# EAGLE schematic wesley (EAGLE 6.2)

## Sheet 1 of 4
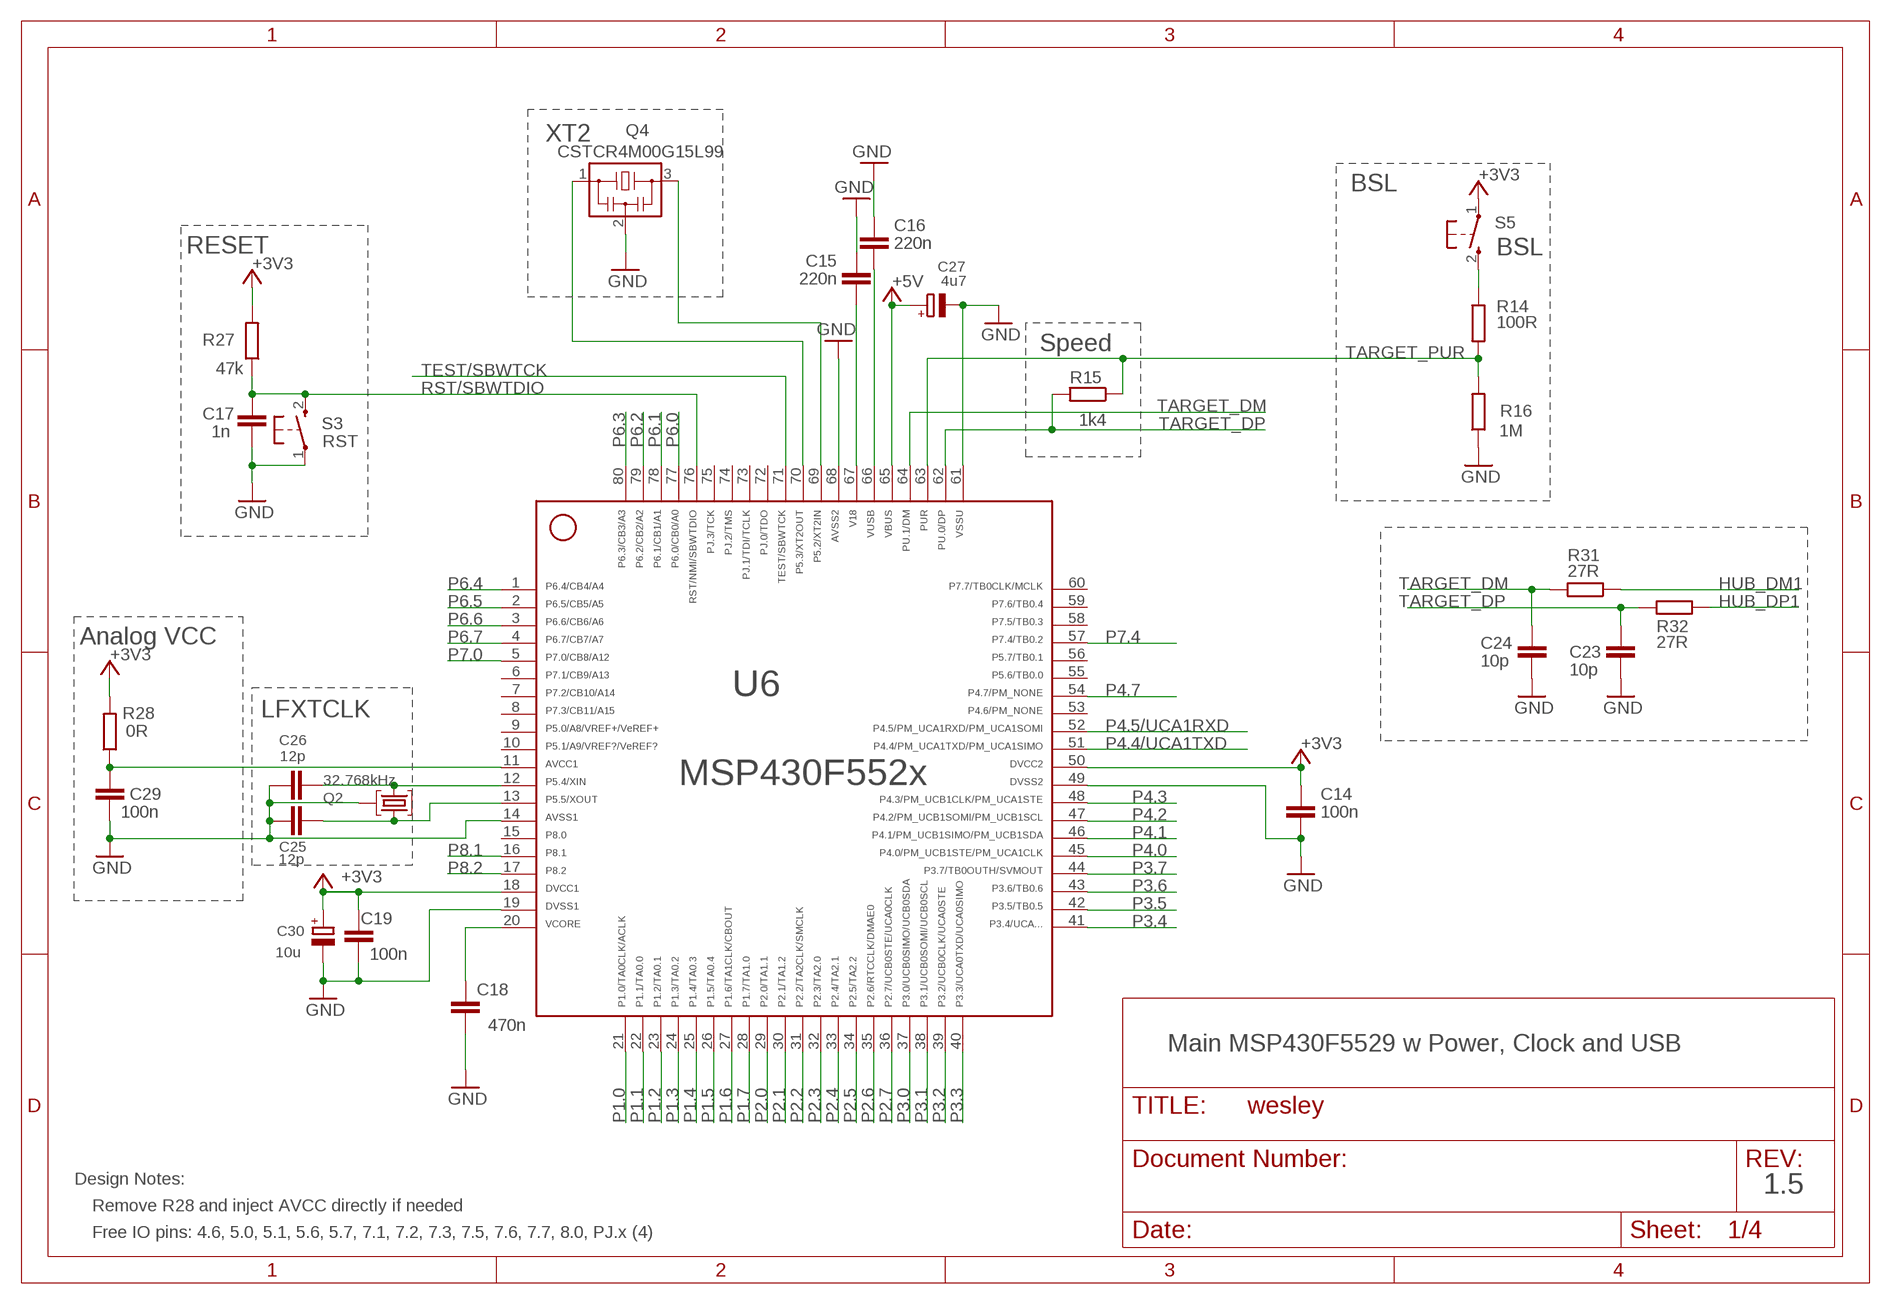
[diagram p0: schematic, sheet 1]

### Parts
C14  100n  C-EUC0402  [C0402]
C15  220n  C-EUC0402  [C0402]
C16  220n  C-EUC0402  [C0402]
C17  1n  C-EUC0402  [C0402]
C18  470n  C-EUC0402  [C0402]
C19  100n  C-EUC0402  [C0402]
C23  10p  C-EUC0402  [C0402]
C24  10p  C-EUC0402  [C0402]
C25  12p  C-EUC0402  [C0402]
C26  12p  C-EUC0402  [C0402]
C27  4u7  CPOL-EUA/3216-18R  [A/3216-18R]
C29  100n  C-EUC0402  [C0402]
C30  10u  CPOL-EUA/3216-18R  [A/3216-18R]
Q2  32.768kHz  MS3V-T1R  [MS3V-T1R]
Q4  CSTCR4M00G15L99  MURATA-FILTER_CSTCR6M00G53Z  [MURATA-FILTER_CSTCR]
R14  100R  R-EU_R0402  [R0402]
R15  1k4  R-EU_R0402  [R0402]
R16  1M  R-EU_R0402  [R0402]
R27  47k  R-EU_R0402  [R0402]
R28  0R  R-EU_R0402  [R0402]
R31  27R  R-EU_R0402  [R0402]
R32  27R  R-EU_R0402  [R0402]
S3  RST  PB  [PBTH]
S5  BSL  PB  [PBTH]
U6  MSP430F5529IPNR  F552X---PN80  [PN80]

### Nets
+3V3 [Power]: C14.1 C19.2 C30.+ R27.2 R28.2 S5.1(P) U6.18 U6.50 ; also sheet 2
+5V [Power]: C27.+ U6.65 ; also sheet 2
AVCC [Power]: C29.1 R28.1 U6.11
GND [Ground]: C14.2 C15.2 C16.2 C17.2 C18.1 C19.1 C23.2 C24.2 C25.1 C26.1 C27.- C29.2 C30.- Q2.P3(GND) Q4.2 R16.1 S3.1(P) U6.14 U6.19 U6.49 U6.61 U6.68 ; also sheet 2,3,4
HUB_DM1: R31.1 ; also sheet 4
HUB_DP1: R32.1 ; also sheet 4
N$4: R14.1 S5.2(S)
P1.0: U6.21 ; also sheet 2
P1.1: U6.22 ; also sheet 2
P1.2: U6.23 ; also sheet 2
P1.3: U6.24 ; also sheet 2
P1.4: U6.25 ; also sheet 2
P1.5: U6.26 ; also sheet 2
P1.6: U6.27 ; also sheet 2
P1.7: U6.28 ; also sheet 2
P2.0: U6.29 ; also sheet 2
P2.1: U6.30 ; also sheet 2
P2.2: U6.31 ; also sheet 2
P2.3: U6.32 ; also sheet 2
P2.4: U6.33 ; also sheet 2
P2.5: U6.34 ; also sheet 2
P2.6: U6.35 ; also sheet 2
P2.7: U6.36 ; also sheet 2
P3.0: U6.37 ; also sheet 2
P3.1: U6.38 ; also sheet 2
P3.2: U6.39 ; also sheet 2
P3.3: U6.40 ; also sheet 2
P3.4: U6.41 ; also sheet 2
P3.5: U6.42 ; also sheet 2
P3.6: U6.43 ; also sheet 2
P3.7: U6.44 ; also sheet 2
P4.0: U6.45 ; also sheet 2
P4.1: U6.46 ; also sheet 2
P4.2: U6.47 ; also sheet 2
P4.3: U6.48 ; also sheet 2
P4.4/UCA1TXD: U6.51 ; also sheet 2
P4.5/UCA1RXD: U6.52 ; also sheet 2
P4.7: U6.54 ; also sheet 2
P5.2/XT2IN: Q4.3 U6.69
P5.3/XT2OUT: Q4.1 U6.70
P5.4/XIN: C26.2 Q2.P2 U6.12
P5.5/XOUT: C25.2 Q2.P1 U6.13
P6.0: U6.77 ; also sheet 2
P6.1: U6.78 ; also sheet 2
P6.2: U6.79 ; also sheet 2
P6.3: U6.80 ; also sheet 2
P6.4: U6.1 ; also sheet 2
P6.5: U6.2 ; also sheet 2
P6.6: U6.3 ; also sheet 2
P6.7: U6.4 ; also sheet 2
P7.0: U6.5 ; also sheet 2
P7.4: U6.57 ; also sheet 2
P8.1: U6.16 ; also sheet 2
P8.2: U6.17 ; also sheet 2
RST/SBWTDIO: C17.1 R27.1 S3.2(S) U6.76 ; also sheet 2
TARGET_DM: C24.1 R31.2 U6.64
TARGET_DP: C23.1 R15.2 R32.2 U6.62
TARGET_PUR: R14.2 R15.1 R16.2 U6.63
TARGET_VUSB [Power]: C16.1 U6.66
TEST/SBWTCK: U6.71 ; also sheet 2
V18 [Power]: C15.1 U6.67
VCORE [Power]: C18.2 U6.20
Unconnected: U6.6 U6.7 U6.8 U6.9 U6.10 U6.15 U6.53 U6.55 U6.56 U6.58 U6.59 U6.60 U6.72 U6.73 U6.74 U6.75

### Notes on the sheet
- XT2
- BSL
- RESET
- Speed
- Analog VCC
- LFXTCLK
- Main MSP430F5529 w Power, Clock and USB
- Design Notes:
- 1.5
- Remove R28 and inject AVCC directly if needed
- Free IO pins: 4.6, 5.0, 5.1, 5.6, 5.7, 7.1, 7.2, 7.3, 7.5, 7.6, 7.7, 8.0, PJ.x (4)

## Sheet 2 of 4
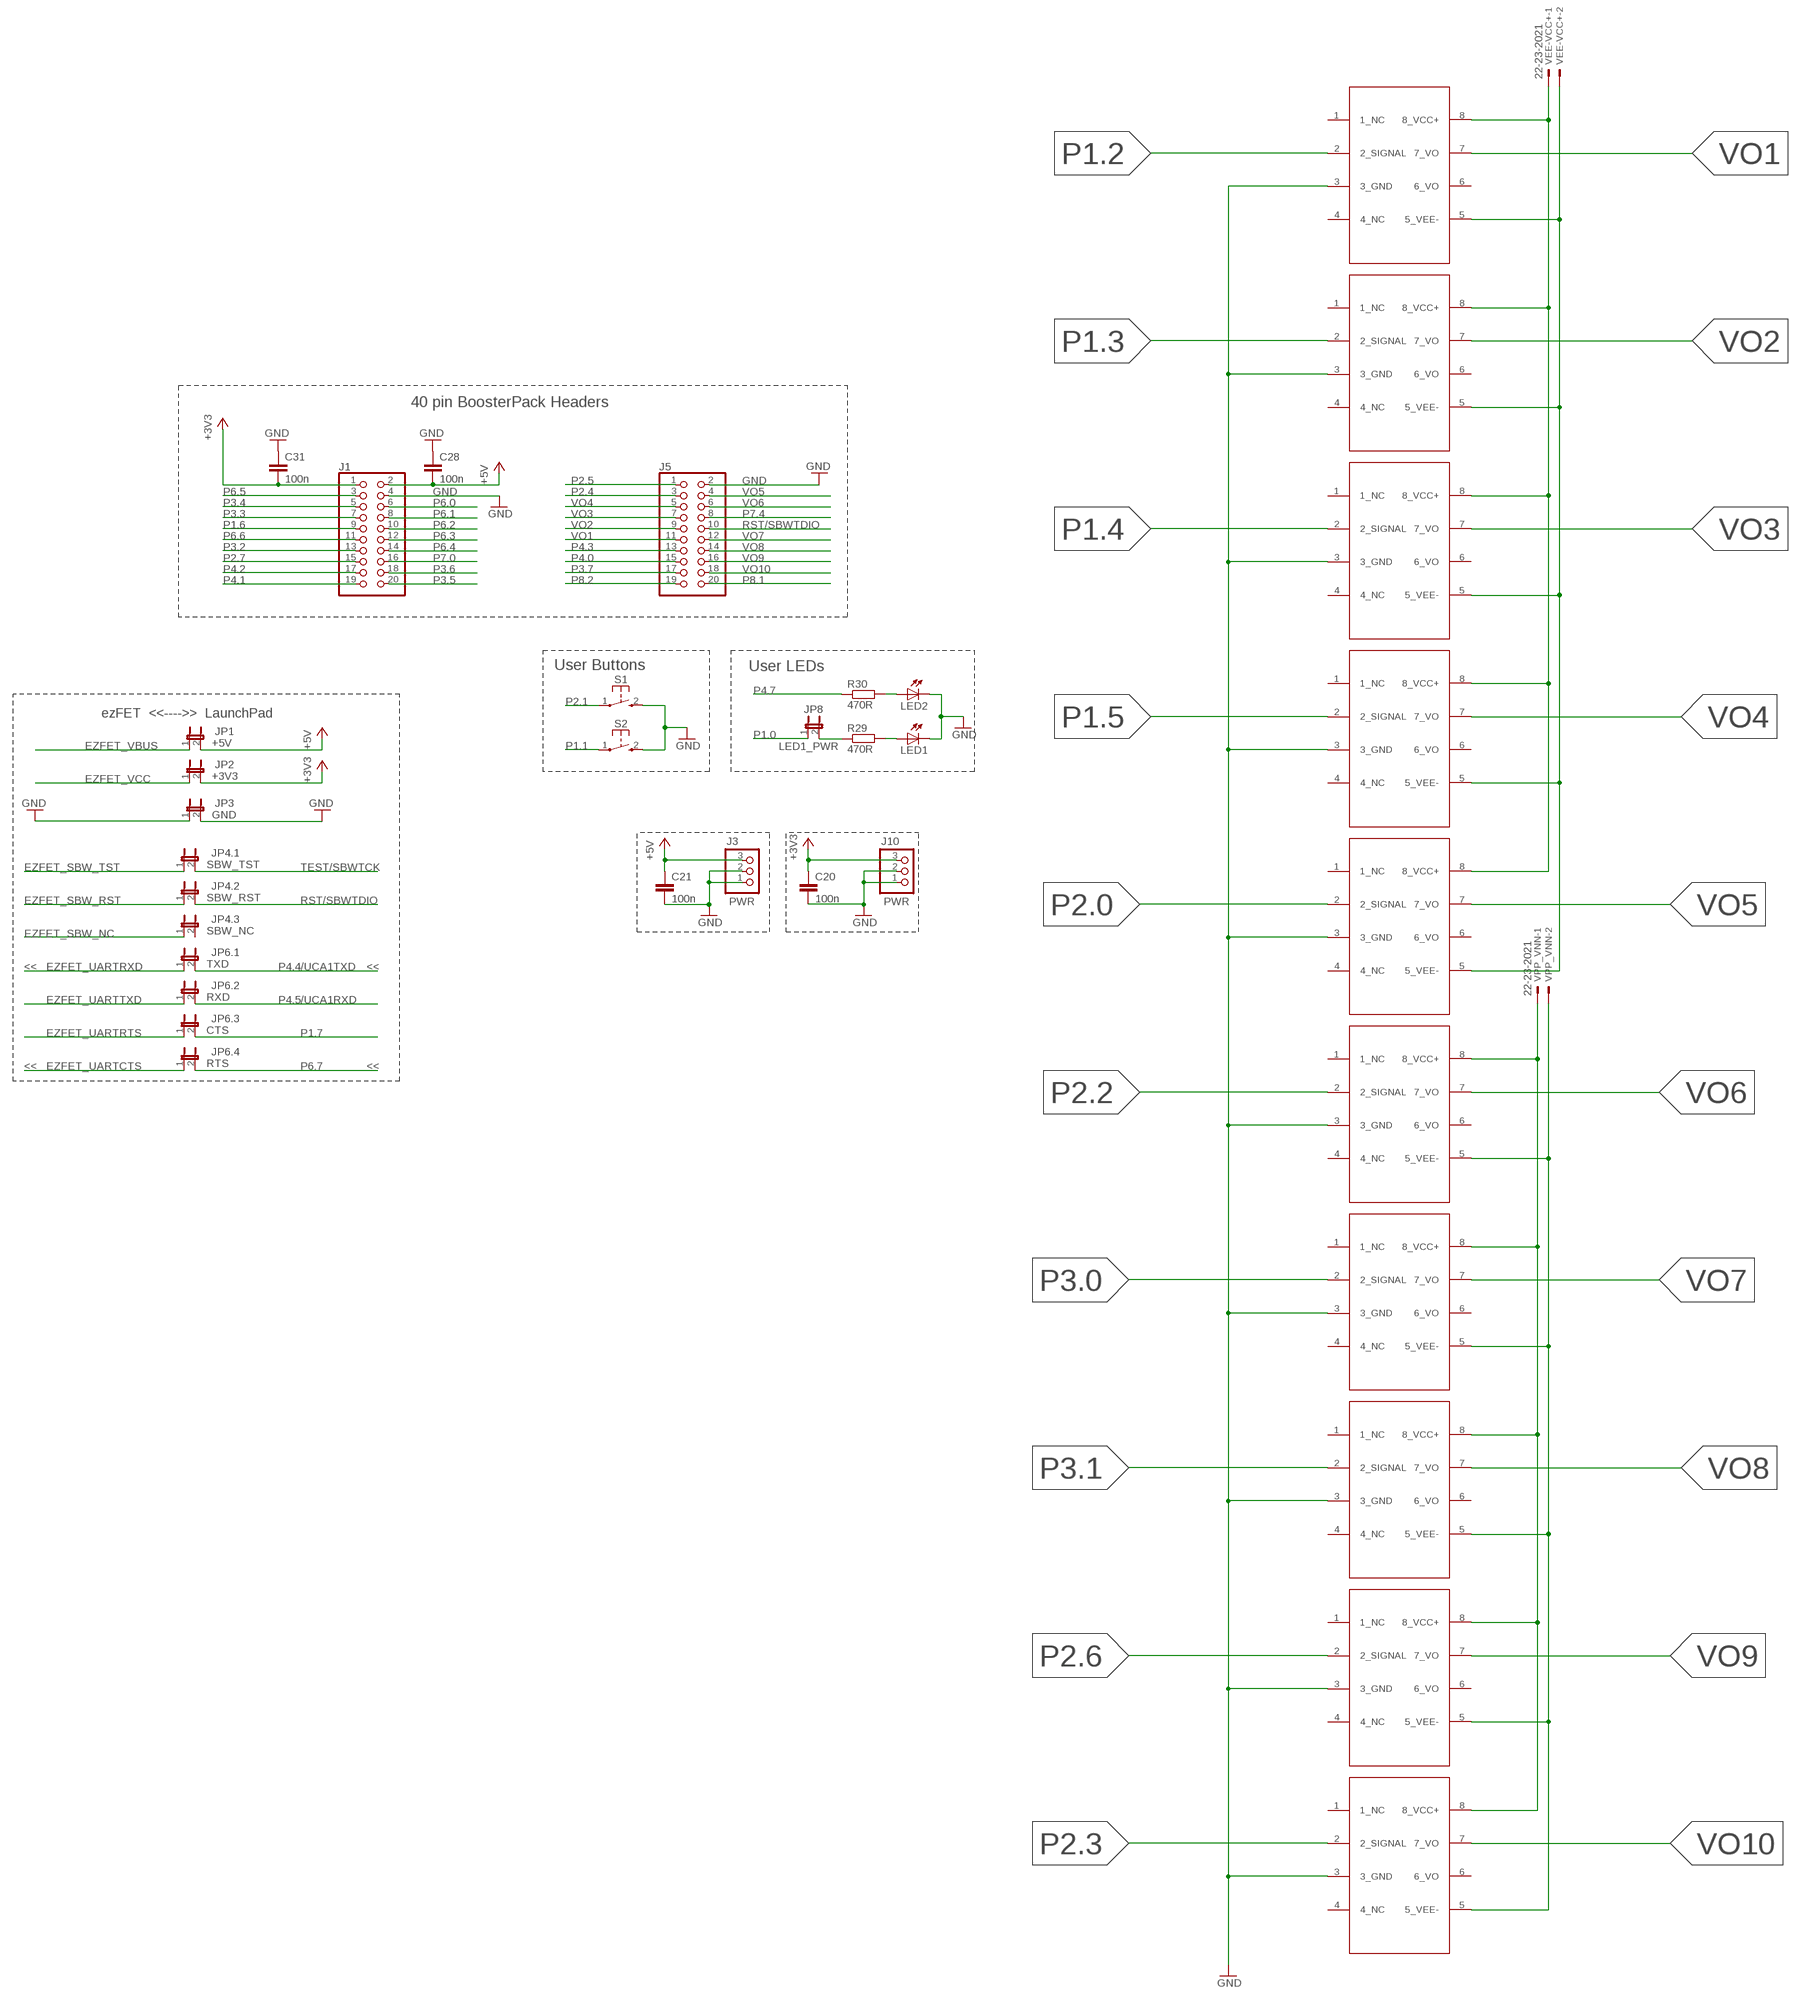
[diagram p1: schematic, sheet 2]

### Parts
C20  100n  C-EUC0402  [C0402]
C21  100n  C-EUC0402  [C0402]
C28  100n  C-EUC0402  [C0402]
C31  100n  C-EUC0402  [C0402]
J1  PINHD-2X10  [2X10]
J3  PWR  PINHD-1X3  [1X03]
J5  PINHD-2X10  [2X10]
J10  PWR  PINHD-1X3  [1X03]
JP1  +5V  JP1M  [JP1M]
JP2  +3V3  JP1M  [JP1M]
JP3  GND  JP1M  [JP1M]
JP4.1  SBW_TST  JP1M  [JP1M]
JP4.2  SBW_RST  JP1M  [JP1M]
JP4.3  SBW_NC  JP1M  [JP1M]
JP6.1  TXD  JP1M  [JP1M]
JP6.2  RXD  JP1M  [JP1M]
JP6.3  CTS  JP1M  [JP1M]
JP6.4  RTS  JP1M  [JP1M]
JP8  LED1_PWR  JP1E  [JP1]
LED1  LEDCHIPLED_0603  [CHIPLED_0603]
LED2  LEDCHIPLED_0603  [CHIPLED_0603]
OPTO1  VO3150A  [8-DIP]
OPTO2  VO3150A  [8-DIP]
OPTO3  VO3150A  [8-DIP]
OPTO4  VO3150A  [8-DIP]
OPTO5  VO3150A  [8-DIP]
OPTO6  VO3150A  [8-DIP]
OPTO7  VO3150A  [8-DIP]
OPTO8  VO3150A  [8-DIP]
OPTO9  VO3150A  [8-DIP]
OPTO10  VO3150A  [8-DIP]
R29  470R  R-EU_R0402  [R0402]
R30  470R  R-EU_R0402  [R0402]
S1  PB  [PBTH]
S2  PB  [PBTH]
VEE-VCC+  22-23-2021  [22-23-2021]
VPP_VNN  22-23-2021  [22-23-2021]

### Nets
+3V3 [Power]: C20.1 C31.2 J1.1 J10.3 JP2.2 ; also sheet 1
+5V [Power]: C21.1 C28.2 J1.2 J3.3 JP1.2 ; also sheet 1
EZFET_SBW_NC: JP4.3.1 ; also sheet 3
EZFET_SBW_RST: JP4.2.1 ; also sheet 3
EZFET_SBW_TST: JP4.1.1 ; also sheet 3
EZFET_UARTCTS: JP6.4.1 ; also sheet 3
EZFET_UARTRTS: JP6.3.1 ; also sheet 3
EZFET_UARTRXD: JP6.1.1 ; also sheet 3
EZFET_UARTTXD: JP6.2.1 ; also sheet 3
EZFET_VBUS [Power]: JP1.1 ; also sheet 3,4
EZFET_VCC [Power]: JP2.1 ; also sheet 3,4
GND [Ground]: C20.2 C21.2 C28.1 C31.1 J1.4 J3.1 J3.2 J5.2 J10.1 J10.2 JP3.1 JP3.2 LED1.C LED2.C OPTO1.3(3_GND) OPTO2.3(3_GND) OPTO3.3(3_GND) OPTO4.3(3_GND) OPTO5.3(3_GND) OPTO6.3(3_GND) OPTO7.3(3_GND) OPTO8.3(3_GND) OPTO9.3(3_GND) OPTO10.3(3_GND) S1.2(S) S2.2(S) ; also sheet 1,3,4
N$7: JP8.2 R29.1
N$32: LED1.A R29.2
N$35: LED2.A R30.2
P1.0: JP8.1 ; also sheet 1
P1.1: S2.1(P) ; also sheet 1
P1.2: OPTO1.2(2_SIGNAL) ; also sheet 1
P1.3: OPTO2.2(2_SIGNAL) ; also sheet 1
P1.4: OPTO3.2(2_SIGNAL) ; also sheet 1
P1.5: OPTO4.2(2_SIGNAL) ; also sheet 1
P1.6: J1.9 ; also sheet 1
P1.7: JP6.3.2 ; also sheet 1
P2.0: OPTO5.2(2_SIGNAL) ; also sheet 1
P2.1: S1.1(P) ; also sheet 1
P2.2: OPTO6.2(2_SIGNAL) ; also sheet 1
P2.3: OPTO10.2(2_SIGNAL) ; also sheet 1
P2.4: J5.3 ; also sheet 1
P2.5: J5.1 ; also sheet 1
P2.6: OPTO9.2(2_SIGNAL) ; also sheet 1
P2.7: J1.15 ; also sheet 1
P3.0: OPTO7.2(2_SIGNAL) ; also sheet 1
P3.1: OPTO8.2(2_SIGNAL) ; also sheet 1
P3.2: J1.13 ; also sheet 1
P3.3: J1.7 ; also sheet 1
P3.4: J1.5 ; also sheet 1
P3.5: J1.20 ; also sheet 1
P3.6: J1.18 ; also sheet 1
P3.7: J5.17 ; also sheet 1
P4.0: J5.15 ; also sheet 1
P4.1: J1.19 ; also sheet 1
P4.2: J1.17 ; also sheet 1
P4.3: J5.13 ; also sheet 1
P4.4/UCA1TXD: JP6.1.2 ; also sheet 1
P4.5/UCA1RXD: JP6.2.2 ; also sheet 1
P4.7: R30.1 ; also sheet 1
P6.0: J1.6 ; also sheet 1
P6.1: J1.8 ; also sheet 1
P6.2: J1.10 ; also sheet 1
P6.3: J1.12 ; also sheet 1
P6.4: J1.14 ; also sheet 1
P6.5: J1.3 ; also sheet 1
P6.6: J1.11 ; also sheet 1
P6.7: JP6.4.2 ; also sheet 1
P7.0: J1.16 ; also sheet 1
P7.4: J5.8 ; also sheet 1
P8.1: J5.20 ; also sheet 1
P8.2: J5.19 ; also sheet 1
RST/SBWTDIO: J5.10 JP4.2.2 ; also sheet 1
TEST/SBWTCK: JP4.1.2 ; also sheet 1
VCC+: OPTO1.8(8_VCC+) OPTO2.8(8_VCC+) OPTO3.8(8_VCC+) OPTO4.8(8_VCC+) OPTO5.8(8_VCC+) VEE-VCC+.1
VEE-: OPTO1.5(5_VEE-) OPTO2.5(5_VEE-) OPTO3.5(5_VEE-) OPTO4.5(5_VEE-) OPTO5.5(5_VEE-) VEE-VCC+.2
VNN-: OPTO6.5(5_VEE-) OPTO7.5(5_VEE-) OPTO8.5(5_VEE-) OPTO9.5(5_VEE-) OPTO10.5(5_VEE-) VPP_VNN.2
VO1: J5.11 OPTO1.7(7_VO)
VO2: J5.9 OPTO2.7(7_VO)
VO3: J5.7 OPTO3.7(7_VO)
VO4: J5.5 OPTO4.7(7_VO)
VO5: J5.4 OPTO5.7(7_VO)
VO6: J5.6 OPTO6.7(7_VO)
VO7: J5.12 OPTO7.7(7_VO)
VO8: J5.14 OPTO8.7(7_VO)
VO9: J5.16 OPTO9.7(7_VO)
VO10: J5.18 OPTO10.7(7_VO)
VPP+: OPTO6.8(8_VCC+) OPTO7.8(8_VCC+) OPTO8.8(8_VCC+) OPTO9.8(8_VCC+) OPTO10.8(8_VCC+) VPP_VNN.1
Unconnected: JP4.3.2 OPTO1.1(1_NC) OPTO1.4(4_NC) OPTO1.6(6_VO) OPTO2.1(1_NC) OPTO2.4(4_NC) OPTO2.6(6_VO) OPTO3.1(1_NC) OPTO3.4(4_NC) OPTO3.6(6_VO) OPTO4.1(1_NC) OPTO4.4(4_NC) OPTO4.6(6_VO) OPTO5.1(1_NC) OPTO5.4(4_NC) OPTO5.6(6_VO) OPTO6.1(1_NC) OPTO6.4(4_NC) OPTO6.6(6_VO) OPTO7.1(1_NC) OPTO7.4(4_NC) OPTO7.6(6_VO) OPTO8.1(1_NC) OPTO8.4(4_NC) OPTO8.6(6_VO) OPTO9.1(1_NC) OPTO9.4(4_NC) OPTO9.6(6_VO) OPTO10.1(1_NC) OPTO10.4(4_NC) OPTO10.6(6_VO)

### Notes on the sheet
- 40 pin BoosterPack Headers
- User Buttons | User LEDs
- ezFET  <<---->>  LaunchPad
- << | <<
- << | <<

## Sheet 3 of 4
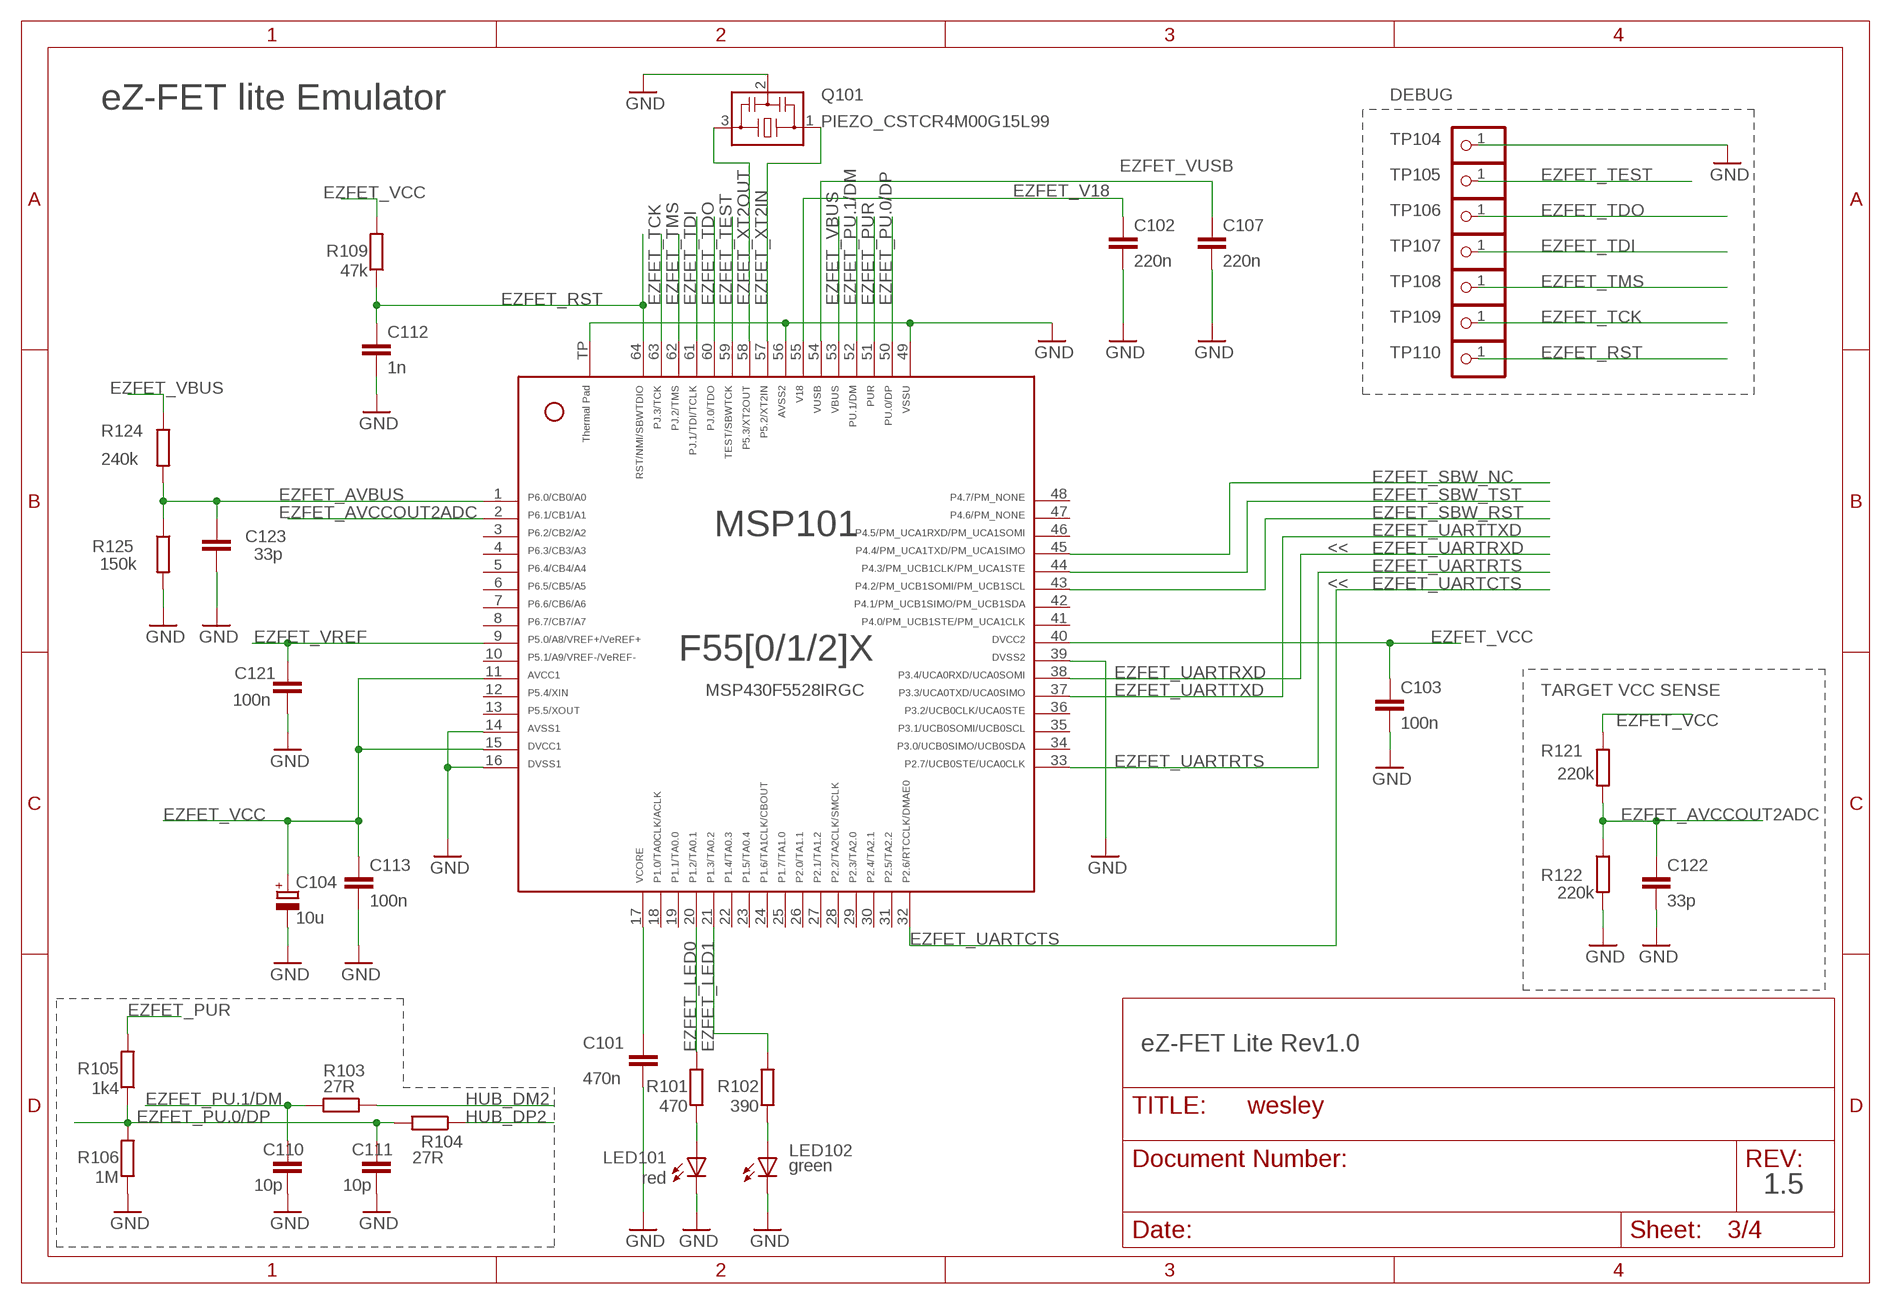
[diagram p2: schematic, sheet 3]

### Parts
C101  470n  C-EUC0402  [C0402]
C102  220n  C-EUC0402  [C0402]
C103  100n  C-EUC0402  [C0402]
C104  10u  CPOL-EUA/3216-18R  [A/3216-18R]
C107  220n  C-EUC0402  [C0402]
C110  10p  C-EUC0402  [C0402]
C111  10p  C-EUC0402  [C0402]
C112  1n  C-EUC0402  [C0402]
C113  100n  C-EUC0402  [C0402]
C121  100n  C-EUC0402  [C0402]
C122  33p  C-EUC0402  [C0402]
C123  33p  C-EUC0402  [C0402]
LED101  red  LEDCHIP-LED0603  [CHIP-LED0603]
LED102  green  LEDCHIP-LED0603  [CHIP-LED0603]
MSP101  MSP430F5528IRGC  F55[0/1/2]X---RGC64  [RGC64]
Q101  PIEZO_CSTCR4M00G15L99  MURATA-FILTER_CSTCR6M00G53Z  [MURATA-FILTER_CSTCR]
R101  470  R-EU_R0402  [R0402]
R102  390  R-EU_R0402  [R0402]
R103  27R  R-EU_R0402  [R0402]
R104  27R  R-EU_R0402  [R0402]
R105  1k4  R-EU_R0402  [R0402]
R106  1M  R-EU_R0402  [R0402]
R109  47k  R-EU_R0402  [R0402]
R121  220k  R-EU_R0402  [R0402]
R122  220k  R-EU_R0402  [R0402]
R124  240k  R-EU_R0402  [R0402]
R125  150k  R-EU_R0402  [R0402]
TP104  TEST_PIN2  PINHD-1X1  [1X01]
TP105  TEST_PIN2  PINHD-1X1  [1X01]
TP106  TEST_PIN2  PINHD-1X1  [1X01]
TP107  TEST_PIN2  PINHD-1X1  [1X01]
TP108  TEST_PIN2  PINHD-1X1  [1X01]
TP109  TEST_PIN2  PINHD-1X1  [1X01]
TP110  TEST_PIN2  PINHD-1X1  [1X01]

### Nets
EZFET_AVBUS: C123.2 MSP101.1 R124.2 R125.1
EZFET_AVCCOUT2ADC: C122.2 MSP101.2 R121.2 R122.1
EZFET_LED0: MSP101.20 R101.2
EZFET_LED1: MSP101.21 R102.2
EZFET_PU.0/DP: C111.1 MSP101.50 R104.2 R105.1 R106.2
EZFET_PU.1/DM: C110.1 MSP101.52 R103.2
EZFET_PUR: MSP101.51 R105.2
EZFET_RST: C112.1 MSP101.64 R109.1 TP110.1
EZFET_SBW_NC: MSP101.45 ; also sheet 2
EZFET_SBW_RST: MSP101.43 ; also sheet 2
EZFET_SBW_TST: MSP101.44 ; also sheet 2
EZFET_TCK: MSP101.63 TP109.1
EZFET_TDI: MSP101.61 TP107.1
EZFET_TDO: MSP101.60 TP106.1
EZFET_TEST: MSP101.59 TP105.1
EZFET_TMS: MSP101.62 TP108.1
EZFET_UARTCTS: MSP101.32 ; also sheet 2
EZFET_UARTRTS: MSP101.33 ; also sheet 2
EZFET_UARTRXD: MSP101.38 ; also sheet 2
EZFET_UARTTXD: MSP101.37 ; also sheet 2
EZFET_V18 [Power]: C102.1 MSP101.55
EZFET_VBUS [Power]: MSP101.53 R124.1 ; also sheet 2,4
EZFET_VCC [Power]: C103.1 C104.+ C113.1 MSP101.11 MSP101.15 MSP101.40 R109.2 R121.1 ; also sheet 2,4
EZFET_VREF [Power]: C121.1 MSP101.9
EZFET_VUSB [Power]: C107.1 MSP101.54
EZFET_XT2IN: MSP101.57 Q101.1
EZFET_XT2OUT: MSP101.58 Q101.3
GND [Ground]: C101.2 C102.2 C103.2 C104.- C107.2 C110.2 C111.2 C112.2 C113.2 C121.2 C122.1 C123.1 LED101.C LED102.C MSP101.14 MSP101.16 MSP101.39 MSP101.49 MSP101.56 MSP101.TP Q101.2 R106.1 R122.2 R125.2 TP104.1 ; also sheet 1,2,4
HUB_DM2: R103.1 ; also sheet 4
HUB_DP2: R104.1 ; also sheet 4
N$1: LED101.A R101.1
N$2: LED102.A R102.1
N$8: C101.1 MSP101.17
Unconnected: MSP101.3 MSP101.4 MSP101.5 MSP101.6 MSP101.7 MSP101.8 MSP101.10 MSP101.12 MSP101.13 MSP101.18 MSP101.19 MSP101.22 MSP101.23 MSP101.24 MSP101.25 MSP101.26 MSP101.27 MSP101.28 MSP101.29 MSP101.30 MSP101.31 MSP101.34 MSP101.35 MSP101.36 MSP101.41 MSP101.42 MSP101.46 MSP101.47 MSP101.48

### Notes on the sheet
- DEBUG
- eZ-FET lite Emulator
- <<
- <<
- MSP430F5528IRGC | TARGET VCC SENSE
- eZ-FET Lite Rev1.0
- 1.5

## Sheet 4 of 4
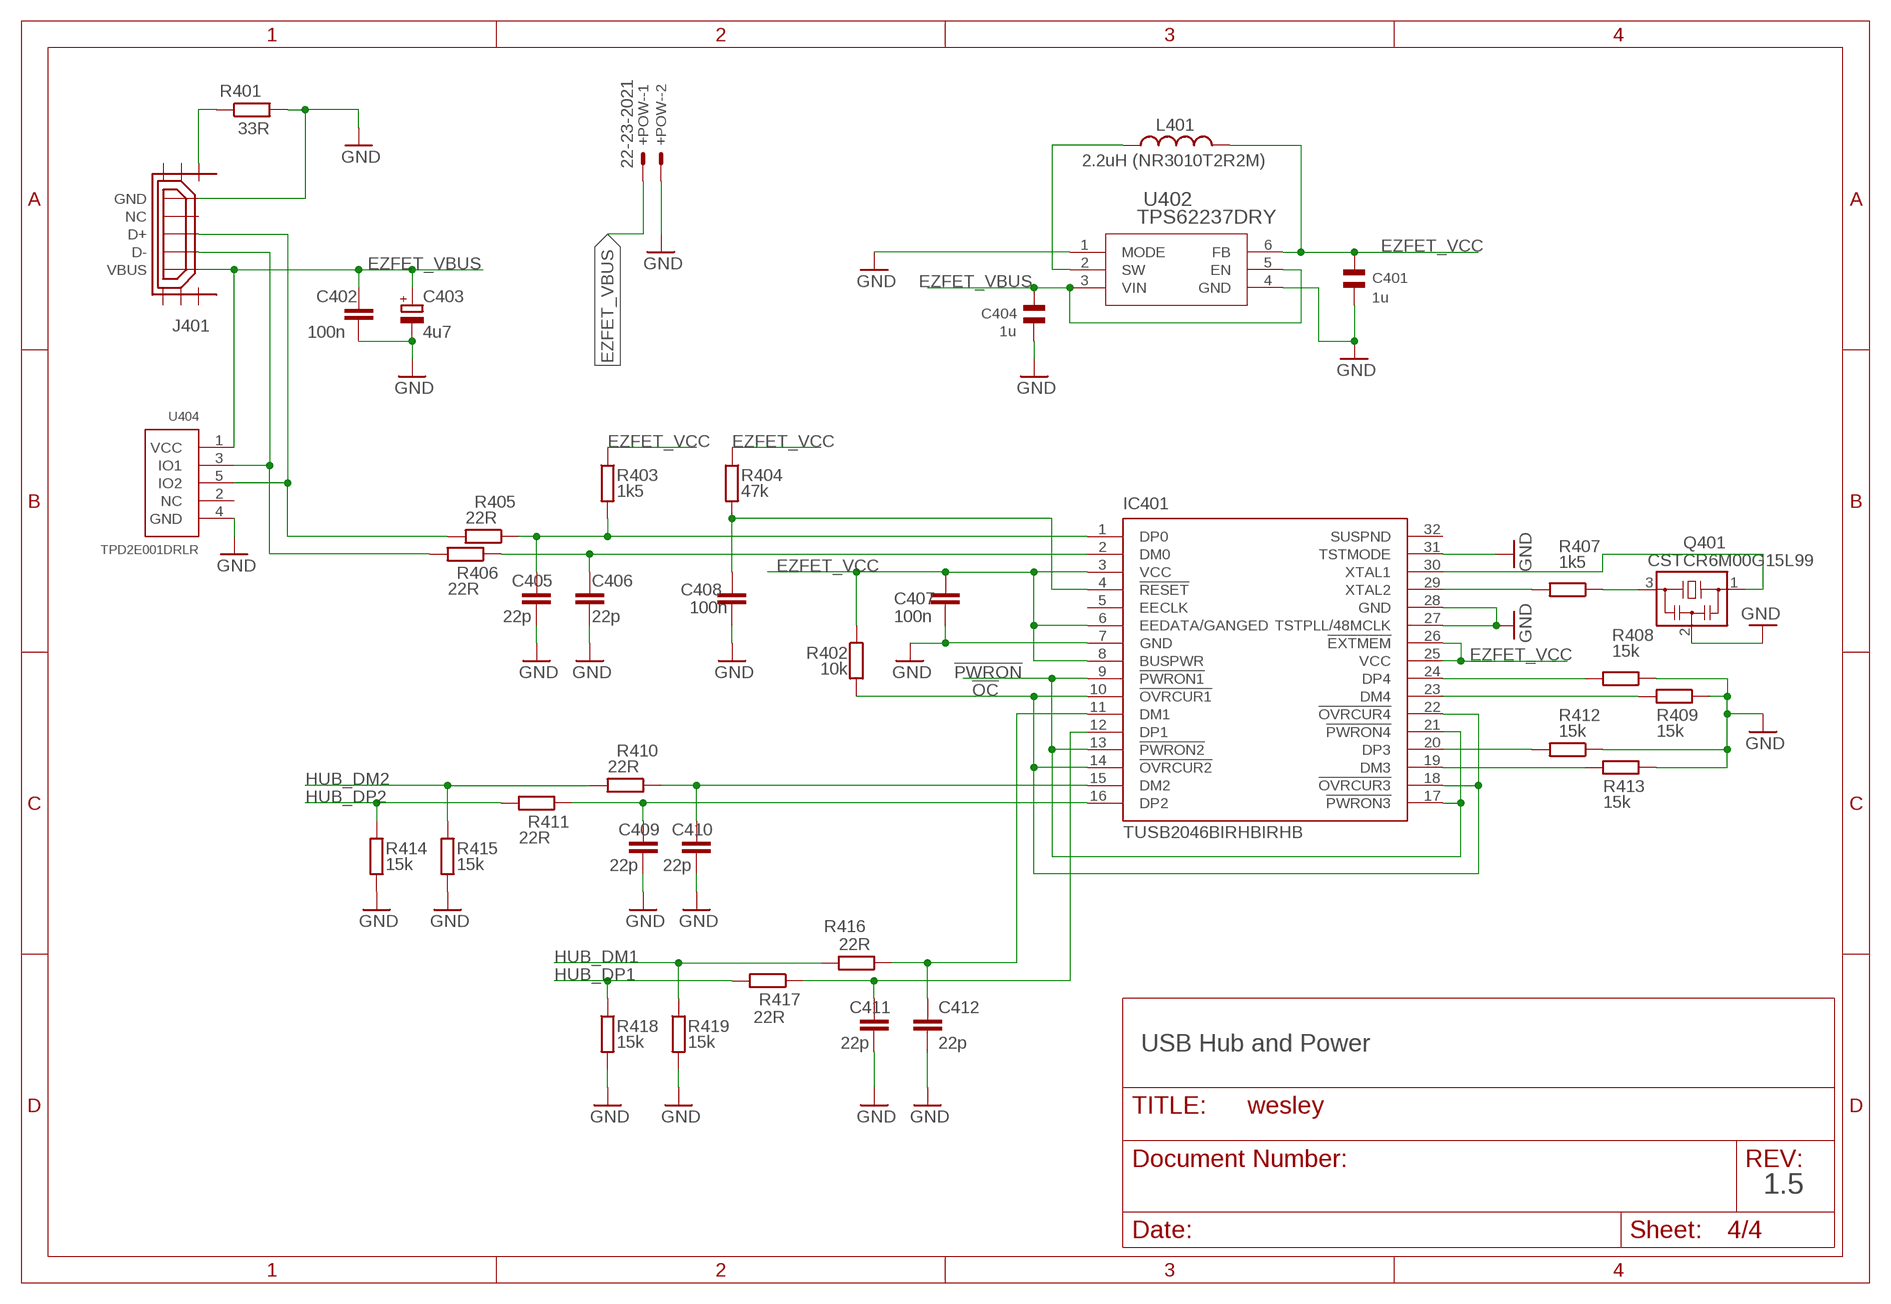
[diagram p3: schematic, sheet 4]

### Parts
+POW-  22-23-2021  [22-23-2021]
C401  1u  CSMD0805  [CSMD0805]
C402  100n  C-EUC0402  [C0402]
C403  4u7  CPOL-EUA/3216-18R  [A/3216-18R]
C404  1u  CSMD0805  [CSMD0805]
C405  22p  C-EUC0402  [C0402]
C406  22p  C-EUC0402  [C0402]
C407  100n  C-EUC0402  [C0402]
C408  100n  C-EUC0402  [C0402]
C409  22p  C-EUC0402  [C0402]
C410  22p  C-EUC0402  [C0402]
C411  22p  C-EUC0402  [C0402]
C412  22p  C-EUC0402  [C0402]
IC401  TUSB2046BIRHBIRHB  [RHB_S-PQFP-N32]
J401  USB_MICRO_FLIPPED  [HIROSE-ZX62R-B-5P]
L401  2.2uH (NR3010T2R2M)  L-NR3010  [L-NR3010]
Q401  CSTCR6M00G15L99  MURATA-FILTER_CSTCR6M00G53Z  [MURATA-FILTER_CSTCR]
R401  33R  R-EU_R0402  [R0402]
R402  10k  R-EU_R0402  [R0402]
R403  1k5  R-EU_R0402  [R0402]
R404  47k  R-EU_R0402  [R0402]
R405  22R  R-EU_R0402  [R0402]
R406  22R  R-EU_R0402  [R0402]
R407  1k5  R-EU_R0402  [R0402]
R408  15k  R-EU_R0402  [R0402]
R409  15k  R-EU_R0402  [R0402]
R410  22R  R-EU_R0402  [R0402]
R411  22R  R-EU_R0402  [R0402]
R412  15k  R-EU_R0402  [R0402]
R413  15k  R-EU_R0402  [R0402]
R414  15k  R-EU_R0402  [R0402]
R415  15k  R-EU_R0402  [R0402]
R416  22R  R-EU_R0402  [R0402]
R417  22R  R-EU_R0402  [R0402]
R418  15k  R-EU_R0402  [R0402]
R419  15k  R-EU_R0402  [R0402]
U402  TPS62237DRY  TPS6223X_DRY_6  [DRY6]
U404  TPD2E001DRLR  TPD2E001  [TPD2E001-DRL]

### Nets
!OC: IC401.10(!OVRCUR1) IC401.14(!OVRCUR2) IC401.18(!OVRCUR3) IC401.22(!OVRCUR4) R402.2
!PWRON: IC401.9(!PWRON1) IC401.13(!PWRON2) IC401.17(!PWRON3) IC401.21(!PWRON4)
EZFET_VBUS [Power]: +POW-.1 C402.1 C403.+ C404.2 J401.VBUS U402.3(VIN) U402.5(EN) U404.1(VCC) ; also sheet 2,3
EZFET_VCC [Power]: C401.2 C407.1 IC401.3(VCC) IC401.6(EEDATA/GANGED) IC401.8(BUSPWR) IC401.25(VCC) IC401.26(!EXTMEM) L401.P$2 R402.1 R403.1 R404.1 U402.6(FB) ; also sheet 2,3
GND [Ground]: +POW-.2 C401.1 C402.2 C403.- C404.1 C405.2 C406.2 C407.2 C408.2 C409.2 C410.2 C411.2 C412.2 IC401.7(GND) IC401.27(TSTPLL/48MCLK) IC401.28(GND) IC401.31(TSTMODE) J401.GND Q401.2 R401.2 R408.1 R409.1 R412.1 R413.1 R414.2 R415.2 R418.2 R419.2 U402.1(MODE) U402.4(GND) U404.4(GND) ; also sheet 1,2,3
HUB_DM1: R416.2 R419.1 ; also sheet 1
HUB_DM2: R410.2 R415.1 ; also sheet 3
HUB_DP1: R417.2 R418.1 ; also sheet 1
HUB_DP2: R411.2 R414.1 ; also sheet 3
N$3: C410.1 IC401.15(DM2) R410.1
N$5: C405.1 IC401.1(DP0) R403.2 R405.1
N$6: IC401.30(XTAL1) Q401.1
N$10: J401.SHIELD1 R401.1
N$11: C406.1 IC401.2(DM0) R406.1
N$12: J401.D+ R405.2 U404.5(IO2)
N$13: J401.D- R406.2 U404.3(IO1)
N$14: L401.P$1 U402.2(SW)
N$15: IC401.29(XTAL2) R407.2
N$16: C412.1 IC401.11(DM1) R416.1
N$17: C411.1 IC401.12(DP1) R417.1
N$18: C409.1 IC401.16(DP2) R411.1
N$19: C408.1 IC401.4(!RESET) R404.2
N$20: IC401.20(DP3) R412.2
N$21: IC401.24(DP4) R408.2
N$22: IC401.23(DM4) R409.2
N$23: IC401.19(DM3) R413.2
N$28: Q401.3 R407.1
Unconnected: IC401.5(EECLK) IC401.32(SUSPND) IC401.EXP IC401.EXP@1(EXP) IC401.EXP@2(EXP) IC401.EXP@3(EXP) IC401.EXP@4(EXP) IC401.EXP@5(EXP) IC401.EXP@6(EXP) IC401.EXP@7(EXP) IC401.EXP@8(EXP) IC401.EXP@9(EXP) J401.NC J401.SHIELD2 J401.SHIELD3 J401.SHIELD4 J401.SHIELD5 J401.SHIELD6 U404.2(NC)

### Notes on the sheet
- USB Hub and Power
- 1.5

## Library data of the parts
+POW- VEE-VCC+ VPP_VNN = con-molex:22-23-2021: .100" (2.54mm) Center Header - 2 Pin; MF: MOLEX; MPN: 22-23-2021; OC_FARNELL: 1462926; OC_NEWARK: 25C3832
C14-C21 C23-C26 C28 C29 C31 C101-C103 C107 C110-C113 C121-C123 C402 C405-C412 = rcl:C-EU: CAPACITOR, European symbol
C27 C30 C104 C403 = rcl:CPOL-EU: POLARIZED CAPACITOR, European symbol
C401 C404 = CAP:CSMD0805
IC401 = texas:TUSB2046BIRHB: 4-PORT HUB FOR THE UNIVERSAL SERIAL BUS WITH OPTIONAL SERIAL EEPROM INTERFACE Source: http://focus.ti.com/lit/ds/symlink/tusb2046b.pdf; MPN: TUSB2046BIRHBT; OC_FARNELL: 1610201; OC_NEWARK: 14N8499
J1 J5 = pinhead:PINHD-2X10: PIN HEADER
J3 J10 = pinhead:PINHD-1X3: PIN HEADER
J401 = usb_con-update:USB_MICRO_FLIPPED
JP1-JP3 JP4.1-JP4.3 JP6.1-JP6.4 = jumper:JP1M
JP8 = jumper:JP1E: JUMPER
L401 = MSP-EXP430F5659:L-NR3010
LED1 LED2 LED101 LED102 = led:LED: LED
MSP101 = TI_MSP430_v16_intern:F55[0/1/2]X---RGC64: ***F55[0/1/2]X***RGC64 Rev. 1.0 06/2010 "http://www.ti.com/lit/gpn/msp430f5529" "http://www.ti.com/lit/gpn/msp430f5509" F5513/F5514 with limited Functions on some Pins
OPTO1-OPTO10 = zoilo:VO3150A
Q2 = microcrystal:MS3V-T1R
Q4 Q101 Q401 = murata:MURATA-FILTER_CSTCR: Resonator Source: murata.co.jp; MPN: CSTCR6M00G53-R0; OC_FARNELL: 1170434; OC_NEWARK: 25M8759
R14-R16 R27-R32 R101-R106 R109 R121 R122 R124 R125 R401-R419 = rcl:R-EU_: RESISTOR, European symbol
S1-S3 S5 = electricalmeter:PB: OMRON SWITCH
TP104-TP110 = pinhead:PINHD-1X1: PIN HEADER
U6 = TI_MSP430_v16_intern:F552X---PN80: ***MSP430F552X***PN80 http://www.ti.com/lit/gpn/msp430f5529 Rev1.0 06/2010 For F552X where X is 1,5,7,9
U402 = tps62231dry:TPS6223X_DRY_6; DATASHEETURL: http://www.ti.com/lit/gpn/TPS62231; DESCRIPTION: 3 MHz Ultra Small Step Down Converter in 1x1.5 SON Package; FAMILY_NAME: STEP-DOWN REGULATOR; GENERIC_PART_NUMBER: TPS62231; INDUSTRY_STD_PKG_TYPE: SON; MANUFACTURER: Texas Instruments; MANUFACTURER_PART_NUMBER: tps62231_dry_6; PACKAGE_DESIGNATOR: DRY; PIN_COUNT: 6; VALUE: TPS6223xDRY; VENDOR: Texas Instuments
U404 = Project7264:TPD2E001: TPD2E001 ESD-protection diode array

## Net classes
0 Default: width 0.203 mm, drill 0.305 mm, clearance 0.152 mm
1 Ground: width 0.203 mm, drill 0.305 mm, clearance 0.152 mm to class 0, clearance 0.152 mm
2 Power: width 0.203 mm, drill 0.305 mm, clearance 0.152 mm to class 0, clearance 0.152 mm to class 1, clearance 0.152 mm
